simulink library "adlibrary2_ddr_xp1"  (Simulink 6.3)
undefined symbols (not defined in the file or in its folder): adlibrary2, ADM, DDR, II, memsize, SDRAM, Simulation, Subsystem, XRC, XRM
libraries: xbsIndex_r4 x29, adlibrary2_ddr_xpl x1, adlibrary2_ddr_xp0 x1

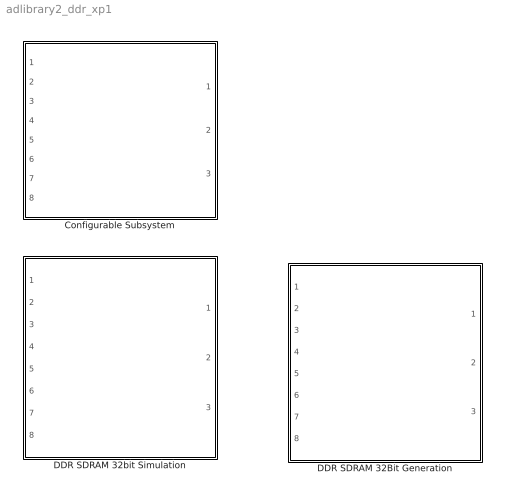
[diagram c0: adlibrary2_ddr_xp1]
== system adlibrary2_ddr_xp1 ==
  Configurable Subsystem : Subsystem  Tag=configX  BlockChoice=DDR SDRAM 32bit Simulation  mask{memsize=memsize}
      mask prompts: memsize "Simulation Ram Size (Mb)"
  DDR SDRAM 32Bit Generation : Subsystem
  DDR SDRAM 32bit Simulation : Subsystem  mask{memsize=memsize}
      mask prompts: memsize "Simulation Ram Size (Mb)"

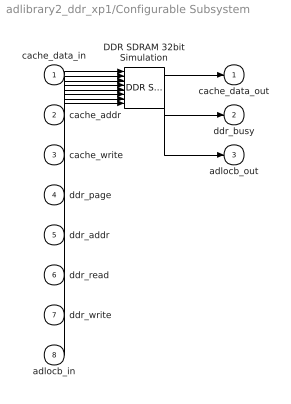
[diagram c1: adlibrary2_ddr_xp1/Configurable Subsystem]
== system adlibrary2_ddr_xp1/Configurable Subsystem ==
  cache_data_in : Inport
  cache_addr : Inport  Port=2
  cache_write : Inport  Port=3
  ddr_page : Inport  Port=4
  ddr_addr : Inport  Port=5
  ddr_read : Inport  Port=6
  ddr_write : Inport  Port=7
  adlocb_in : Inport  Port=8
  DDR SDRAM 32bit Simulation : adlibrary2_ddr_xpl/DDR SDRAM 32bit Simulation  memsize=memsize
  cache_data_out : Outport
  ddr_busy : Outport  Port=2
  adlocb_out : Outport  Port=3
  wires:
  cache_data_in/1 -> DDR SDRAM 32bit Simulation/1
  cache_addr/1 -> DDR SDRAM 32bit Simulation/2
  cache_write/1 -> DDR SDRAM 32bit Simulation/3
  ddr_page/1 -> DDR SDRAM 32bit Simulation/4
  ddr_addr/1 -> DDR SDRAM 32bit Simulation/5
  ddr_read/1 -> DDR SDRAM 32bit Simulation/6
  ddr_write/1 -> DDR SDRAM 32bit Simulation/7
  adlocb_in/1 -> DDR SDRAM 32bit Simulation/8
  DDR SDRAM 32bit Simulation/1 -> cache_data_out/1
  DDR SDRAM 32bit Simulation/2 -> ddr_busy/1
  DDR SDRAM 32bit Simulation/3 -> adlocb_out/1

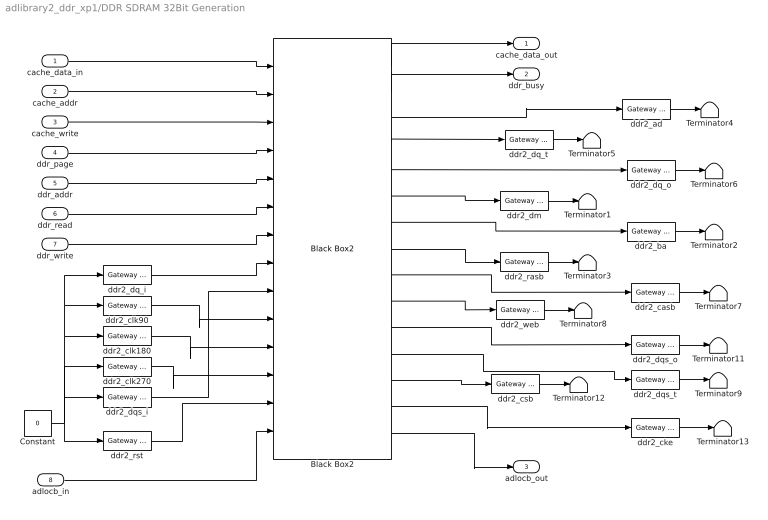
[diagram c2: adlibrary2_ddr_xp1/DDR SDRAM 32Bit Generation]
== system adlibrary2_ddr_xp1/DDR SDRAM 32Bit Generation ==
  cache_data_in : Inport
  cache_addr : Inport  Port=2
  cache_write : Inport  Port=3
  ddr_page : Inport  Port=4
  ddr_addr : Inport  Port=5
  ddr_read : Inport  Port=6
  ddr_write : Inport  Port=7
  adlocb_in : Inport  Port=8
  Black Box2 : adlibrary2_ddr_xp0/DDR SDRAM 32Bit Generation/Black Box2  init_code=ddr32xp_config  sim_method=Inactive  block_type=blackbox2  adlocb_devid=5  ddr_size=64
  Constant : Constant  Value=0
  Terminator{1..9,11..13} (12 alike) : Terminator
  ddr2_ad : xbsIndex_r4/Gateway Out  hdl_port=on  timing_constraint=None  locs_specified=off  LOCs={}  block_type=gatewayout
  ddr2_ba : xbsIndex_r4/Gateway Out  hdl_port=on  timing_constraint=None  locs_specified=off  LOCs={}  block_type=gatewayout
  ddr2_casb : xbsIndex_r4/Gateway Out  hdl_port=on  timing_constraint=None  locs_specified=off  LOCs={}  block_type=gatewayout
  ddr2_cke : xbsIndex_r4/Gateway Out  hdl_port=on  timing_constraint=None  locs_specified=off  LOCs={}  block_type=gatewayout
  ddr2_clk180 : xbsIndex_r4/Gateway In  arith_type=Boolean  n_bits=64  bin_pt=0  period=1  dbl_ovrd=off  timing_constraint=None  locs_specified=off  LOCs={}  block_type=gatewayin
  ddr2_clk270 : xbsIndex_r4/Gateway In  arith_type=Boolean  n_bits=64  bin_pt=0  period=1  dbl_ovrd=off  timing_constraint=None  locs_specified=off  LOCs={}  block_type=gatewayin
  ddr2_clk90 : xbsIndex_r4/Gateway In  arith_type=Boolean  n_bits=64  bin_pt=0  period=1  dbl_ovrd=off  timing_constraint=None  locs_specified=off  LOCs={}  block_type=gatewayin
  ddr2_csb : xbsIndex_r4/Gateway Out  hdl_port=on  timing_constraint=None  locs_specified=off  LOCs={}  block_type=gatewayout
  ddr2_dm : xbsIndex_r4/Gateway Out  hdl_port=on  timing_constraint=None  locs_specified=off  LOCs={}  block_type=gatewayout
  ddr2_dq_i : xbsIndex_r4/Gateway In  arith_type=Unsigned  n_bits=32  bin_pt=0  period=1  dbl_ovrd=off  timing_constraint=None  locs_specified=off  LOCs={}  block_type=gatewayin
  ddr2_dq_o : xbsIndex_r4/Gateway Out  hdl_port=on  timing_constraint=None  locs_specified=off  LOCs={}  block_type=gatewayout
  ddr2_dq_t : xbsIndex_r4/Gateway Out  hdl_port=on  timing_constraint=None  locs_specified=off  LOCs={}  block_type=gatewayout
  ddr2_dqs_i : xbsIndex_r4/Gateway In  arith_type=Unsigned  n_bits=4  bin_pt=0  period=1  dbl_ovrd=off  timing_constraint=None  locs_specified=off  LOCs={}  block_type=gatewayin
  ddr2_dqs_o : xbsIndex_r4/Gateway Out  hdl_port=on  timing_constraint=None  locs_specified=off  LOCs={}  block_type=gatewayout
  ddr2_dqs_t : xbsIndex_r4/Gateway Out  hdl_port=on  timing_constraint=None  locs_specified=off  LOCs={}  block_type=gatewayout
  ddr2_rasb : xbsIndex_r4/Gateway Out  hdl_port=on  timing_constraint=None  locs_specified=off  LOCs={}  block_type=gatewayout
  ddr2_rst : xbsIndex_r4/Gateway In  arith_type=Boolean  n_bits=64  bin_pt=0  period=1  dbl_ovrd=off  timing_constraint=None  locs_specified=off  LOCs={}  block_type=gatewayin
  ddr2_web : xbsIndex_r4/Gateway Out  hdl_port=on  timing_constraint=None  locs_specified=off  LOCs={}  block_type=gatewayout
  cache_data_out : Outport
  ddr_busy : Outport  Port=2
  adlocb_out : Outport  Port=3
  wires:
  Black Box2/15 -> adlocb_out/1
  Black Box2/14 -> ddr2_cke/1
  Black Box2/13 -> ddr2_csb/1
  Black Box2/12 -> ddr2_dqs_t/1
  Black Box2/11 -> ddr2_dqs_o/1
  Black Box2/10 -> ddr2_web/1
  Black Box2/9 -> ddr2_casb/1
  Black Box2/8 -> ddr2_rasb/1
  Black Box2/7 -> ddr2_ba/1
  Black Box2/6 -> ddr2_dm/1
  Black Box2/5 -> ddr2_dq_o/1
  Black Box2/4 -> ddr2_dq_t/1
  Black Box2/3 -> ddr2_ad/1
  ddr2_dqs_t/1 -> Terminator9/1
  Constant/1 -> ddr2_dqs_i/1, ddr2_clk270/1, ddr2_clk180/1, ddr2_clk90/1, ddr2_dq_i/1, ddr2_rst/1
  ddr2_dq_i/1 -> Black Box2/8
  cache_data_in/1 -> Black Box2/1
  cache_addr/1 -> Black Box2/2
  cache_write/1 -> Black Box2/3
  ddr_page/1 -> Black Box2/4
  ddr_addr/1 -> Black Box2/5
  ddr_read/1 -> Black Box2/6
  ddr_write/1 -> Black Box2/7
  Black Box2/1 -> cache_data_out/1
  Black Box2/2 -> ddr_busy/1
  ddr2_ad/1 -> Terminator4/1
  ddr2_dq_t/1 -> Terminator5/1
  ddr2_dq_o/1 -> Terminator6/1
  ddr2_dm/1 -> Terminator1/1
  ddr2_ba/1 -> Terminator2/1
  ddr2_rasb/1 -> Terminator3/1
  ddr2_casb/1 -> Terminator7/1
  ddr2_web/1 -> Terminator8/1
  ddr2_dqs_o/1 -> Terminator11/1
  ddr2_csb/1 -> Terminator12/1
  ddr2_cke/1 -> Terminator13/1
  ddr2_dqs_i/1 -> Black Box2/9
  ddr2_clk90/1 -> Black Box2/10
  ddr2_clk180/1 -> Black Box2/11
  ddr2_clk270/1 -> Black Box2/12
  adlocb_in/1 -> Black Box2/14
  ddr2_rst/1 -> Black Box2/13

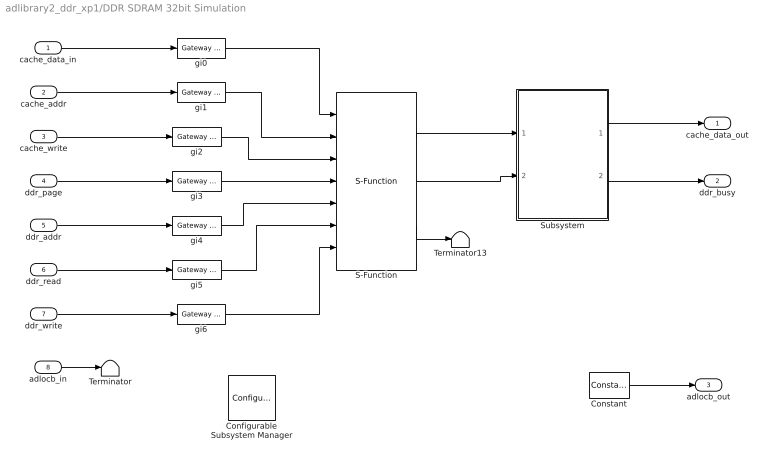
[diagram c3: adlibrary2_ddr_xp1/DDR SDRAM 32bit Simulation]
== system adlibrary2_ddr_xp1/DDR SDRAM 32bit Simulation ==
  cache_data_in : Inport
  cache_addr : Inport  Port=2
  cache_write : Inport  Port=3
  ddr_page : Inport  Port=4
  ddr_addr : Inport  Port=5
  ddr_read : Inport  Port=6
  ddr_write : Inport  Port=7
  adlocb_in : Inport  Port=8
  Configurable Subsystem Manager : xbsIndex_r4/Configurable Subsystem Manager  Tag=xcfgMgr  block_type=configsubsys
  Constant : xbsIndex_r4/Constant  arith_type=Unsigned  const=0  n_bits=66  bin_pt=0  explicit_period=on  period=1  equ=P=C  opselect=C  inp2=PCIN>>17  opr=+  inp1=P  carry=CIN  dbl_ovrd=off  block_type=constant
  S-Function : S-Function  FunctionName=ddr32  Parameters=memsize,0
  Subsystem : Subsystem  AncestorBlock=adlibrary2/ADM-XRC-II/XRM DDR SDRAM /DDR SDRAM 64bit Simulation/Subsystem
  Terminator : Terminator
  Terminator13 : Terminator
  gi{0..6} (7 alike) : xbsIndex_r4/Gateway Out  hdl_port=off  timing_constraint=None  locs_specified=off  LOCs={}  block_type=gatewayout
  cache_data_out : Outport
  ddr_busy : Outport  Port=2
  adlocb_out : Outport  Port=3
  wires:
  cache_data_in/1 -> gi0/1
  cache_addr/1 -> gi1/1
  cache_write/1 -> gi2/1
  ddr_page/1 -> gi3/1
  ddr_addr/1 -> gi4/1
  ddr_read/1 -> gi5/1
  ddr_write/1 -> gi6/1
  gi0/1 -> S-Function/1
  gi1/1 -> S-Function/2
  gi2/1 -> S-Function/3
  gi3/1 -> S-Function/4
  gi4/1 -> S-Function/5
  gi5/1 -> S-Function/6
  gi6/1 -> S-Function/7
  S-Function/2 -> Subsystem/2(In2)
  S-Function/1 -> Subsystem/1(In1)
  Subsystem/1(Out1) -> cache_data_out/1
  Subsystem/2(Out2) -> ddr_busy/1
  S-Function/3 -> Terminator13/1
  Constant/1 -> adlocb_out/1
  adlocb_in/1 -> Terminator/1

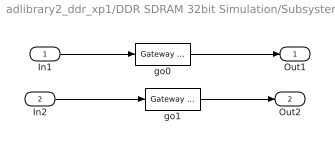
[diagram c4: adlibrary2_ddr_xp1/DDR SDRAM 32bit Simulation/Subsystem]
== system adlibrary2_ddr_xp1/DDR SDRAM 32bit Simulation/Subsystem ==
  In1 : Inport
  In2 : Inport  Port=2
  go0 : xbsIndex_r4/Gateway In  arith_type=Unsigned  n_bits=32  bin_pt=0  period=1  dbl_ovrd=off  timing_constraint=None  locs_specified=off  LOCs={}  block_type=gatewayin
  go1 : xbsIndex_r4/Gateway In  arith_type=Boolean  n_bits=32  bin_pt=0  period=1  dbl_ovrd=off  timing_constraint=None  locs_specified=off  LOCs={}  block_type=gatewayin
  Out1 : Outport
  Out2 : Outport  Port=2
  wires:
  go1/1 -> Out2/1
  go0/1 -> Out1/1
  In2/1 -> go1/1
  In1/1 -> go0/1
